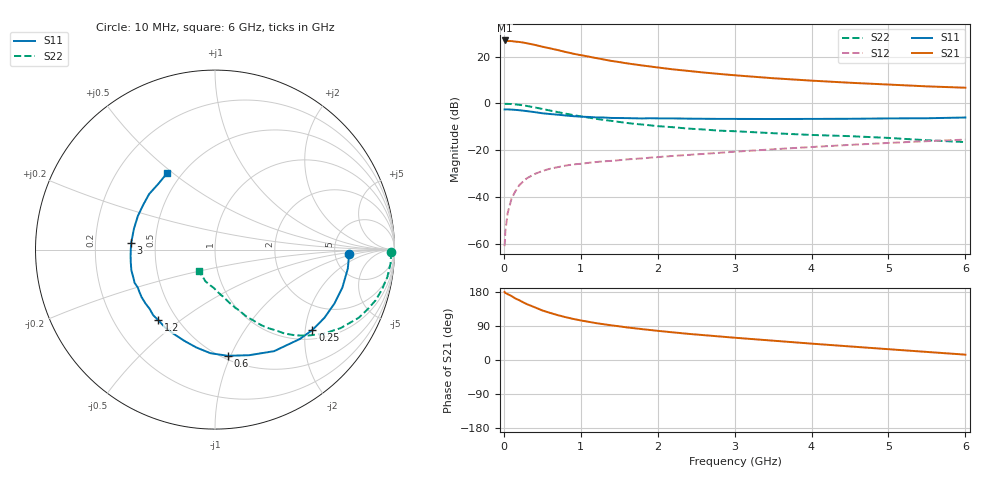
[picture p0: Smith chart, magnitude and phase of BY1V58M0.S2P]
! SIEMENS Small Signal Semiconductors
! BFY420
! Si NPN RF SIEGET Grounded Emitter Transistor in MICRO-X
! VCE = 1.5 V  IC = 8 mA
! Common Emitter S-Parameters:  October  1996
# GHz  S  MA  R  50
!  f  S11  S21  S12  S22
! GHz  MAG  ANG  MAG  ANG  MAG  ANG  MAG  ANG
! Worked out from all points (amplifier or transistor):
!   36 points, 10 MHz to 6 GHz, reference 50 ohm
!   highest |S21| = 26.9 dB at 10 MHz (marker M1)
!   |S21| within 3 dB of that: start of sweep to 548 MHz
!   unconditionally stable (mu >= 1): 2.645 GHz to end of sweep
!   at 250 MHz: K = 0.15, MSG = 29.7 dB, |S12| = -33.4 dB
!   at 1.4 GHz: K = 0.69, MSG = 21.3 dB, |S12| = -24.5 dB
!   at 6 GHz: K = 1.12, MAG = 9.0 dB, |S12| = -15.4 dB
!   S11 on the Smith chart (normalised r, x): 10 MHz: 6.81, -0.68; 250 MHz: 1.23, -2.19; 600 MHz: 0.53, -0.97; 1.2 GHz: 0.40, -0.42; 3 GHz: 0.36, +0.03; 6 GHz: 0.42, +0.47
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0.01  0.7463 -1.7  22.16 179.6  0.0009 96.6  0.9805 -0.7
0.02  0.747 -3.4  22.1 177.0  0.0019 92.7  0.9814 -1.6
0.05  0.7474 -8.2  21.55 173.7  0.0046 90.3  0.9811 -4.4
0.1  0.7406 -16.6  21.48 168.8  0.0093 83.3  0.9724 -9.0
0.15  0.7302 -24.3  20.9 162.3  0.0134 78.2  0.9565 -13.4
0.2  0.7185 -31.9  20.58 157.8  0.018 74.8  0.9386 -17.5
0.25  0.7037 -39.5  20 152.3  0.0215 71.0  0.9115 -21.6
0.3  0.6867 -46.5  19.3 147.4  0.0254 67.8  0.8861 -25.4
0.4  0.6547 -59.8  17.87 139.3  0.0312 62.5  0.8254 -32.0
0.5  0.6186 -72.0  16.31 130.8  0.0362 57.7  0.7648 -37.8
0.6  0.5959 -83.2  15.04 124.4  0.0405 54.5  0.7072 -42.6
0.8  0.5549 -100.9  12.61 113.2  0.0471 49.4  0.6078 -50.3
0.9  0.5367 -108.4  11.59 108.5  0.0501 47.8  0.5667 -52.8
1.1  0.5159 -122.5  10.04 100.8  0.0541 45.7  0.4992 -58.1
1.2  0.5044 -128.8  9.321 97.3  0.0563 45.0  0.4702 -60.2
1.6  0.4872 -147.2  7.191 86.0  0.0641 43.1  0.3844 -66.8
2.2  0.4802 -166.0  5.351 72.9  0.076 41.9  0.3115 -74.3
3  0.4684 175.5  4.003 58.8  0.0935 39.8  0.2559 -82.3
3.5  0.4664 165.5  3.462 51.0  0.1053 38.0  0.2322 -87.2
4.5  0.4715 147.7  2.771 35.8  0.1307 32.3  0.2007 -97.8
5.5  0.4841 130.4  2.32 21.3  0.1569 24.6  0.1642 -115.3
6  0.5022 122.3  2.171 14.1  0.1694 20.5  0.15 -127.2
